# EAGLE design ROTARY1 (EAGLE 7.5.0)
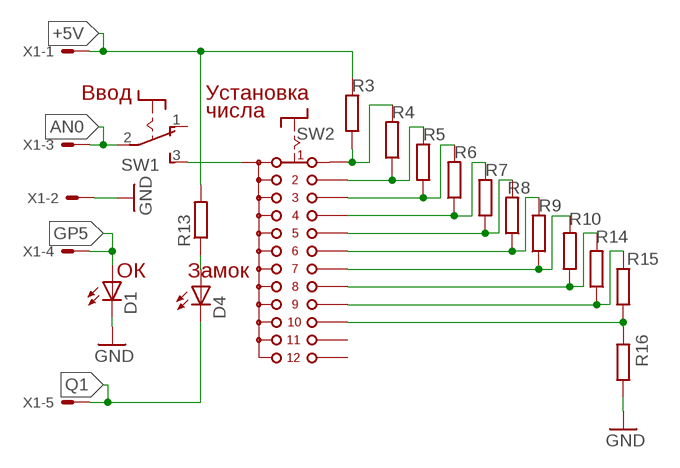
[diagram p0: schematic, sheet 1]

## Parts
D1  LED5MM  [LED5MM]
D4  LED5MM  [LED5MM]
R3  R-EU_M1206  [M1206]
R4  R-EU_M1206  [M1206]
R5  R-EU_M1206  [M1206]
R6  R-EU_M1206  [M1206]
R7  R-EU_M1206  [M1206]
R8  R-EU_M1206  [M1206]
R9  R-EU_M1206  [M1206]
R10  R-EU_M1206  [M1206]
R13  R-EU_M1206  [M1206]
R14  R-EU_M1206  [M1206]
R15  R-EU_M1206  [M1206]
R16  R-EU_M1206  [M1206]
SW1  8MS9P1  [8MS9]
SW2  CK1049  CK101X12  [CK101X12]
X1  22-23-2051  [22-23-2051]

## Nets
+5V: R3.2 R13.2 X1.1
AN0: SW1.2(P) X1.3
GND: D1.K(C) R16.1 X1.2
GP5: D1.A X1.4
N$1: SW1.3(S) SW2.A
N$3: R3.1 R4.2 SW2.1
N$4: R4.1 R5.2 SW2.2
N$5: R5.1 R6.2 SW2.3
N$6: R6.1 R7.2 SW2.4
N$7: R7.1 R8.2 SW2.5
N$8: R14.1 R15.2 SW2.9
N$9: R8.1 R9.2 SW2.6
N$10: R15.1 R16.2 SW2.10
N$12: R9.1 R10.2 SW2.7
N$13: R10.1 R14.2 SW2.8
N$14: D4.A R13.1
Q1: D4.K(C) X1.5
Unconnected: SW1.1(O) SW2.11 SW2.12

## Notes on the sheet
- Ввод | Установка
- числа
- ОК | Замок

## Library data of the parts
D1 D4 = led:LED: LED
R3-R10 R13-R16 = rcl:R-EU_: RESISTOR, European symbol
SW1 = switch:8MS9P1
SW2 = switch:CK101X12: ROTARY SWITCH C&K
X1 = con-molex:22-23-2051: .100" (2.54mm) Center Header - 5 Pin; MF: MOLEX; MPN: 22-23-2051; OC_FARNELL: 1462952; OC_NEWARK: 38C9178

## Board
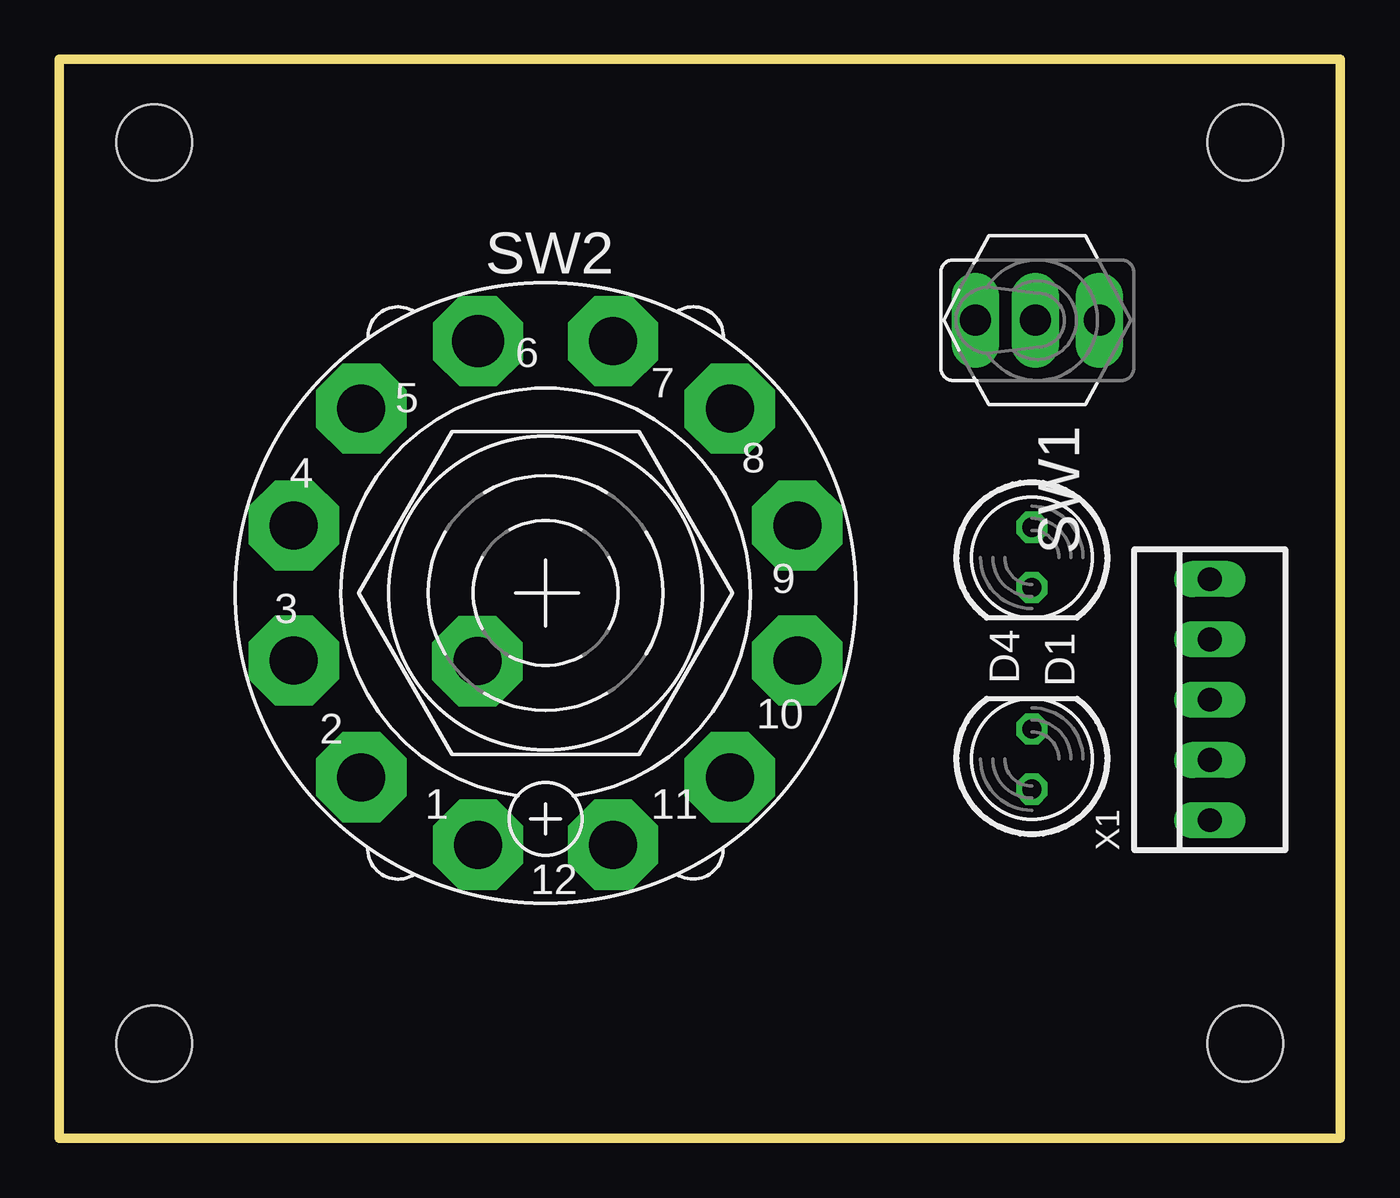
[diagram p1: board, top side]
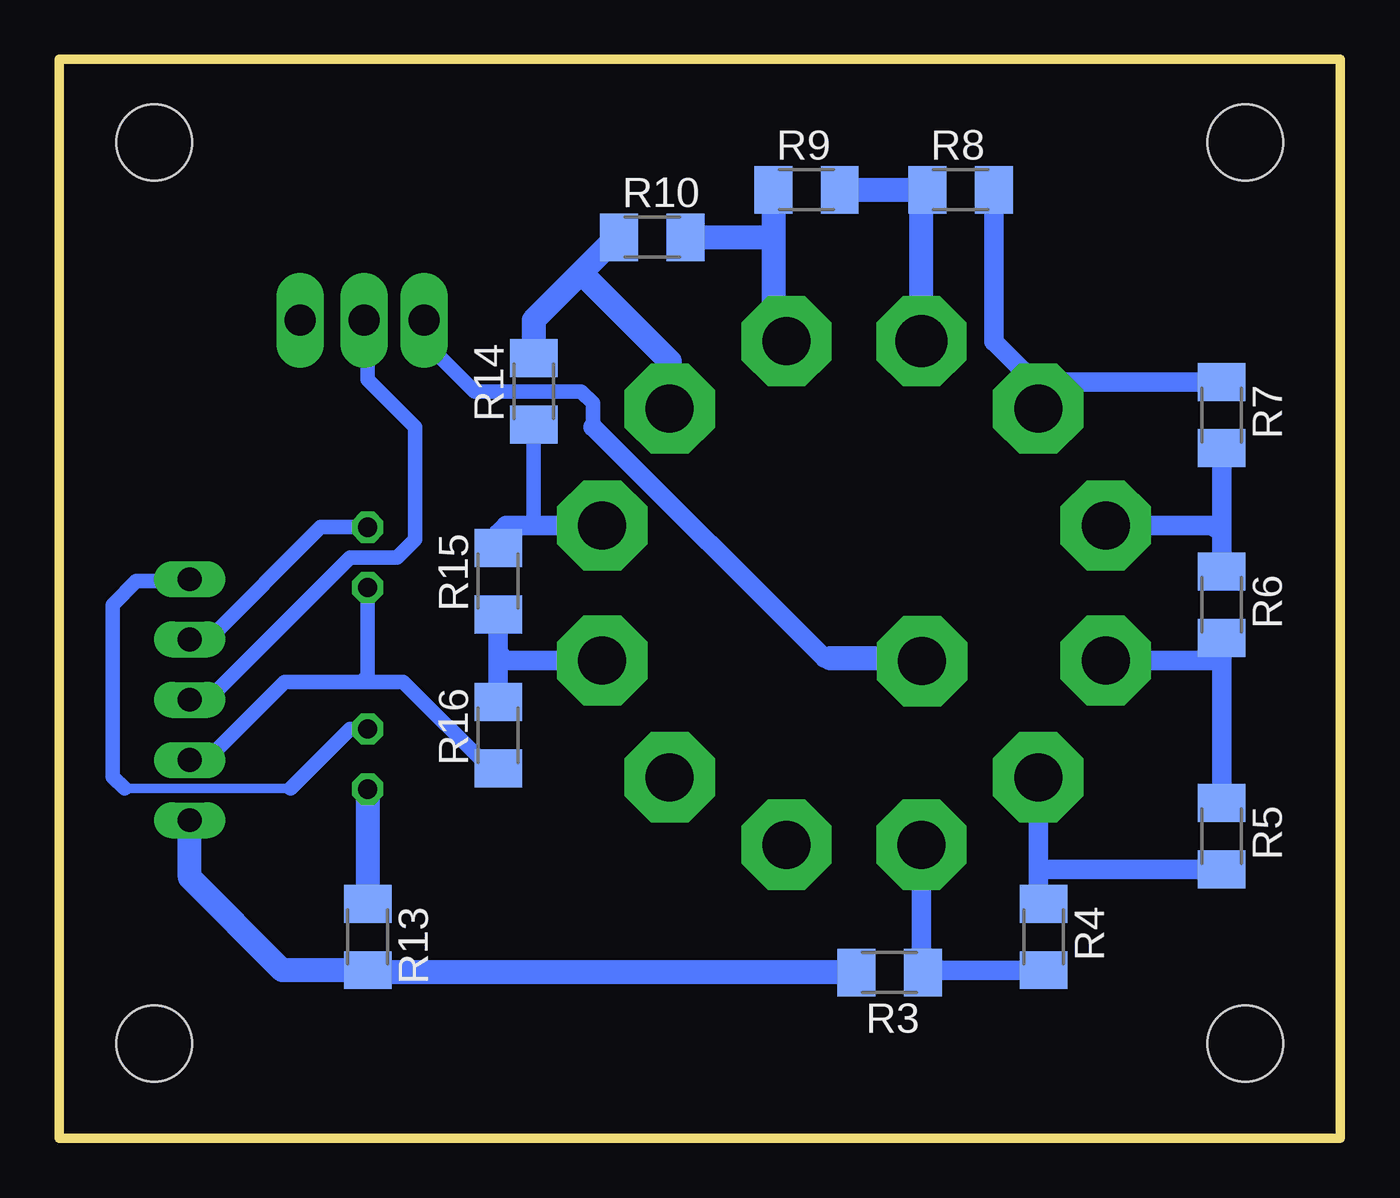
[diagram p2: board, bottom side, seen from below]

Size 54 x 45.5 mm. Coordinates in mm from the lower left corner, seen from the top.
Outline: 0,0 0,45.5 54,45.5 54,0 0,0
Copper layers (1*16): Top 0.035mm / dielectric 1.5mm / Bottom 0.035mm
Design rules "default": minimum track width 10mil, minimum drill 24mil, track to track 8mil, track to pad 8mil, pad to pad 8mil, via to via 8mil, smd to smd 8mil, copper to edge 40mil, drill to drill 8mil, minimum pad ring 10mil, minimum via ring 8mil, stop-mask expansion 4mil, vias tented up to drill 0mil, thermal gap 10mil
Holes 3.2 mm at 4,42 50,42 4,4 50,4

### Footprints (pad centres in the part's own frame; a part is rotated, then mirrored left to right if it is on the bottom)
LED5MM = drill 0.813 octagon: A -1.27,0; K 1.27,0
M1206 = smd 1.6 x 2: 1 -1.4,0; 2 1.4,0
8MS9 = drill 1.295 pad 2 long: 1 -3,5.346 | drill 1.3 pad 2 long: 2 -3,2.654; 3 -3,0.114
CK101X12 = drill 2.032 pad 3.81 octagon: 1 -2.845,-10.617; 2 -7.772,-7.772; 3 -10.617,-2.845; 4 -10.617,2.845; 5 -7.772,7.772; 7 2.845,10.617; 8 7.772,7.772; 9 10.617,2.845; 10 10.617,-2.845; 11 7.772,-7.772; 12 2.845,-10.617; A -2.87,-2.87 | drill 2.2 pad 3.81 octagon: 6 -2.845,10.617
22-23-2051 = drill 1 long: 1 -5.08,0; 2 -2.54,0; 3 0,0; 4 2.54,0; 5 5.08,0

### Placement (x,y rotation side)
D1  41,24.5 270 top
D4  41,16 90 top
R3  19,7 180 bottom
R4  12.5,8.5 270 bottom
R5  5,12.75 270 bottom
R6  5,22.5 270 bottom
R7  5,30.5 270 bottom
R8  16,40 0 bottom
R9  22.5,40 0 bottom
R10  29,38 0 bottom
R13  41,8.5 270 bottom
R14  34,31.5 90 bottom
R15  35.5,23.5 90 bottom
R16  35.5,17 90 bottom
SW1  38.5,31.5 270 top
SW2  20.5,23 0 top
X1  48.5,18.5 90 top

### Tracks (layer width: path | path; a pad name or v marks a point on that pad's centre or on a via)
+5V
  Bottom 1.016: R3.2 40.9,7 R13.2 44.6,7.1 48.5,11 X1.1
AN0
  Bottom 0.61: X1.3 47.75,18.5 41.75,24.5 39.75,24.5 39,25.25 39,30 41,32 41,34.35 SW1.2
GND
  Bottom 0.61: R16.1 35.85,15.6 39.5,19.25 41.25,19.25 | 41.25,19.25 44.5,19.25 47.5,16.25 48.21,16.25 X1.2 | D1.K 41,19.5 41.25,19.25
GP5
  Bottom 0.61: D1.A 42.98,25.77 47.75,21 48.46,21 X1.4
N$1
  Bottom 0.61: SW1.3 38.61,33.61 36.5,31.5 32,31.5 31.5,31 31.5,30 | 21.5,20.25 21.75,20.25
  Bottom 0.813: 21.75,20.25 31.5,30
  Bottom 1.016: 21.5,20.25 17.75,20.25 SW2.A
N$3
  Bottom 0.813: R4.2 17,7.1 | 17,7.1 17.5,7.1 R3.1 | SW2.1 17.66,7.75 17,7.1
N$4
  Bottom 0.813: SW2.2 12.73,11.5 | 12.73,11.5 12.73,10.13 R4.1 | R5.2 12.58,11.35 12.73,11.5
N$5
  Bottom 0.813: R6.2 5,20.5 | 5,20.5 R5.1 | SW2.3 5.34,20.16 5,20.5
N$6
  Bottom 0.813: R6.1 5,25.5 | 5,25.5 R7.2 | SW2.4 5.34,25.84 5,25.5
N$7
  Bottom 0.813: R7.1 11.6,31.9 12.25,31.25 | 12.25,31.25 SW2.5 | R8.2 14.6,33.6 12.25,31.25
N$8
  Bottom 0.61: R14.1 34,26.09 34.25,25.84
  Bottom 0.813: R15.2 35.5,25.5 35.16,25.84 34.25,25.84 SW2.9
N$9
  Bottom 1.016: R9.2 R8.1 17.66,39.74 SW2.6
N$10
  Bottom 0.813: R16.2 35.5,20.5 | 35.5,20.5 R15.1 | SW2.10 35.16,20.16 35.5,20.5
N$12
  Bottom 1.016: R9.1 23.9,38 | 23.9,38 23.9,34.17 SW2.7 | R10.2 23.9,38
N$13
  Bottom 1.016: R10.1 30.5,38 32,36.5 | 32,36.5 34,34.5 R14.2 | SW2.8 28.27,32.77 32,36.5
N$14
  Bottom 1.016: D4.A R13.1
Q1
  Bottom 0.406: 44.25,14.75 51.25,14.75
  Bottom 0.61: D4.K 41.73,17.27 44.25,14.75 | 51.25,14.75 51.75,15.25 51.75,22.5 50.75,23.5 48.58,23.5 X1.5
